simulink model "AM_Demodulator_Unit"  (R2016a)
settings: Solver=ode3  StartTime=0.0  StopTime=1  FixedStep=1/5000000  RelTol=1e-3
libraries: dsparch4 x1

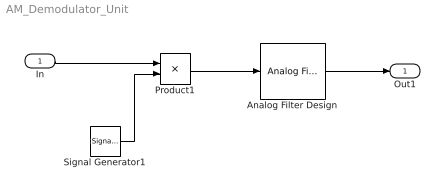
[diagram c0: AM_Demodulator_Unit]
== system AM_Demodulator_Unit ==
  In : Inport
  Analog Filter Design : dsparch4/Analog Filter Design  method=Butterworth  filttype=Lowpass  N=8  Wlo=45000*2*pi  Whi=80  Rp=2  Rs=40
  Product1 : Product
  Signal Generator1 : SignalGenerator  Frequency=500000
  Out1 : Outport
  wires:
  Signal Generator1/1 -> Product1/2
  Analog Filter Design/1 -> Out1/1
  Product1/1 -> Analog Filter Design/1
  In/1 -> Product1/1
